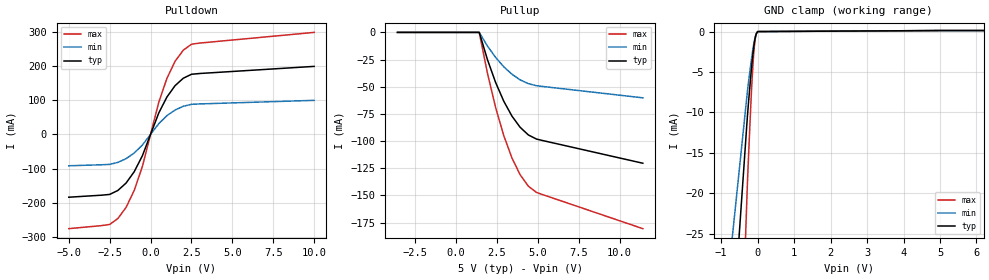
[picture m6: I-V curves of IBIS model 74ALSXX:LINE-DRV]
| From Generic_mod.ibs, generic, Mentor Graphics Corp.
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[Model]   74ALSXX:LINE-DRV
Model_type   I/O
Polarity   Non-Inverting
Vinl  =   0.800V
Vinh  =   2.000V
Vmeas =   1.500V
Cref  =  50.000pF
Rref  =   1.000kOhm
Vref  =   0.000V
|   typ   min   max
C_comp   10.000pF   5.000pF   15.000pF
[Voltage Range]   5.000V   4.500V   5.500V
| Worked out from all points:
|   slope of the pulldown table from 0 to 0.75 V, typ, clamps not added: 8.73 ohm
|   GND clamp passes 1 mA (typ) near -0.08 V on its own axis
[Pulldown]
| Voltage   I(typ)   I(min)   I(max)
-5V       -184mA     -91.98mA   -275.9mA
-2.5V     -175.8mA   -87.88mA   -263.6mA
-2V       -164.2mA   -82.09mA   -246.3mA
-1.5V     -142.6mA   -71.3mA    -213.9mA
-1V       -109.3mA   -54.66mA   -164mA
-500mV    -62.5mA    -31.25mA   -93.75mA
500mV     62.5mA     31.25mA    93.75mA
1V        109.3mA    54.66mA    164mA
1.5V      142.6mA    71.3mA     213.9mA
2V        164.2mA    82.09mA    246.3mA
3V        178mA      89.01mA    267mA
10V       198.8mA    99.42mA    298.3mA
[Pullup]
| Voltage   I(typ)   I(min)   I(max)
-3.577V   0A         0A         0A
1.423V    0A         0A         0A
1.923V    -25mA      -12.5mA    -37.5mA
2.423V    -46.05mA   -23.03mA   -69.08mA
2.923V    -63.35mA   -31.67mA   -95.02mA
3.423V    -77.06mA   -38.53mA   -115.6mA
3.923V    -87.34mA   -43.67mA   -131mA
4.423V    -94.33mA   -47.17mA   -141.5mA
4.923V    -98.19mA   -49.09mA   -147.3mA
11.42V    -120.4mA   -60.21mA   -180.6mA
[GND Clamp]
| Voltage   I(typ)   I(min)   I(max)
-5V       -318.8mA   -213.1mA   -635.1mA
-281.2mV  -10.55mA   -7.454mA   -18.94mA
-248.8mV  -8.731mA   -6.23mA    -15.38mA
-183.3mV  -5.282mA   -3.89mA    -8.735mA
-150.9mV  -3.74mA    -2.827mA   -5.86mA
-120.5mV  -2.458mA   -1.924mA   -3.58mA
-89.36mV  -1.382mA   -1.139mA   -1.82mA
-60.69mV  -665uA     -581.2uA   -789.4uA
-34.72mV  -259.8uA   -239.6uA   -285.2uA
0V        0A         0A         0A
10V       128uA      128uA      128uA
[Ramp]
|   typ   min   max
dV/dt_r   1.485V/2.400ns   0.948V/4.320ns   1.900V/1.760ns
dV/dt_f   2.551V/1.800ns   1.924V/3.240ns   2.973V/1.320ns
R_load =  50.000Ohm
|------------------- End of 74ALSXX:LINE-DRV ----------------------------------
